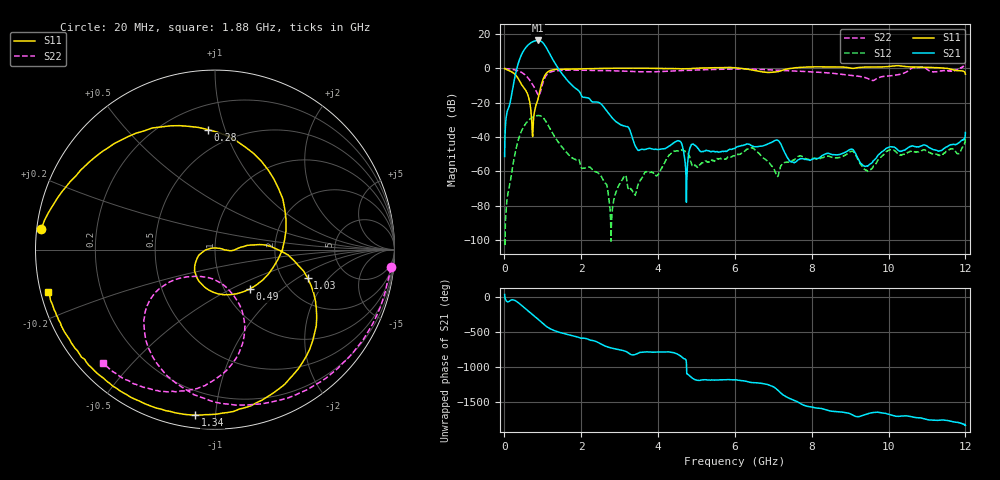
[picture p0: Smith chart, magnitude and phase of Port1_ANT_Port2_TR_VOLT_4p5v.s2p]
! Created Mon Aug 25 11:25:18 2025
# hz S ma R 50
! 2 Port Network Data from SP1.SP block
! freq  magS11  angS11  magS21  angS21  magS12  angS12  magS22  angS22
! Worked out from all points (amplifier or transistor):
!   1200 points, 10 MHz to 12 GHz, reference 50 ohm
!   highest |S21| = 16.2 dB at 870 MHz (marker M1)
!   |S21| within 3 dB of that: 604.8 MHz to 1.062 GHz (457.4 MHz wide, 54.9 % of centre)
!   unconditionally stable (mu >= 1): start of sweep to 2.671 GHz; 3.949 GHz to 4.98 GHz; 6.17 GHz to 7.451 GHz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
!   at 2.01 GHz: K = 42.05, MAG = 1.8 dB, |S12| = -58.0 dB
!   at 6.01 GHz: K = -234.27, MSG = 2.0 dB, |S12| = -50.4 dB
!   at 12 GHz: K = -1645.12, MSG = 1.4 dB, |S12| = -40.3 dB
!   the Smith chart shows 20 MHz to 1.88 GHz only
!   S11 on the Smith chart (normalised r, x): 20 MHz: 0.01, +0.06; 280 MHz: 0.36, +0.87; 490 MHz: 1.30, -0.63; 1.03 GHz: 2.73, -1.23; 1.34 GHz: 0.07, -0.89; 1.88 GHz: 0.02, -0.13
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1e7  0.9818 176.4  0.002698 28.6  1.056e-05 175.0  0.99 -3.2
2e7  0.9744 173.1  0.01025 -16.8  6.597e-06 -119.2  0.985 -5.7
2.8e8  0.6699 93.5  0.5805 -55.9  0.003238 157.3  0.9023 -71.0
3.8e8  0.4715 36.7  1.563 -92.3  0.009148 118.5  0.8322 -93.8
4.9e8  0.2926 -48.9  3.068 -142.5  0.0185 67.8  0.7158 -116.4
5.8e8  0.2064 -111.0  4.28 176.5  0.02633 27.3  0.5881 -132.1
6.6e8  0.1094 -154.5  5.222 140.8  0.0326 -7.8  0.458 -142.3
7.7e8  0.04028 5.3  6.146 91.5  0.03914 -55.9  0.2946 -143.8
8.7e8  0.1185 1.4  6.487 45.8  0.04216 -100.3  0.1777 -122.8
9.5e8  0.2808 5.3  6.21 6.7  0.04105 -138.3  0.2225 -72.8
1.03e9  0.5405 -17.1  5.177 -32.9  0.03475 -176.8  0.4576 -68.6
1.17e9  0.8316 -60.1  2.812 -88.0  0.0194 130.3  0.7452 -92.8
1.34e9  0.9288 -96.8  1.298 -129.4  0.009118 92.7  0.8482 -112.1
1.88e9  0.9587 -165.7  0.2498 152.3  0.002161 46.4  0.8855 -134.7
2.01e9  0.9604 -174.1  0.1599 129.4  0.00126 26.0  0.885 -136.8
2.79e9  1.003 174.1  0.03824 -9.1  2.854e-05 116.0  0.8545 -148.6
4.01e9  0.995 177.2  0.0043 -65.9  0.0008049 56.5  0.8007 142.1
6.01e9  1.035 145.8  0.00474 -99.0  0.003013 -41.2  0.9522 125.0
8.01e9  1.101 71.1  0.002248 -125.8  0.002379 -97.0  0.7871 141.6
1.001e10  1.136 -176.4  0.00504 132.0  0.004118 131.2  0.6008 103.7
1.099e10  1.068 -137.2  0.005585 58.8  0.004039 48.7  0.9599 66.2
1.2e10  0.6767 -71.5  0.01346 -26.1  0.0097 -53.6  1.339 -171.9
